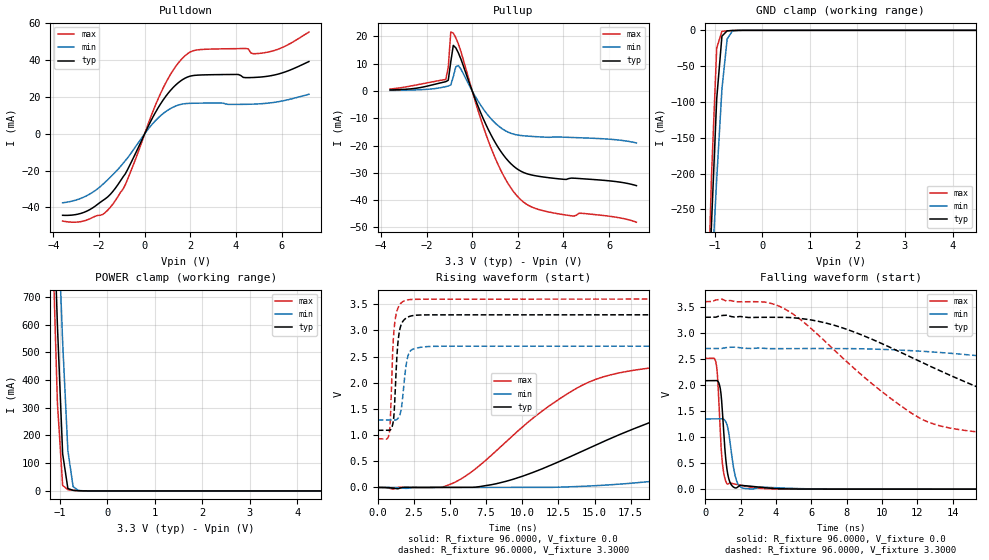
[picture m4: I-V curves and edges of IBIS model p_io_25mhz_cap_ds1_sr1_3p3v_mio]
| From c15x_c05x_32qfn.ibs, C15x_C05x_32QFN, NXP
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[Model] p_io_25mhz_cap_ds1_sr1_3p3v_mio
|   Model p_io_25mhz_cap_ds1_sr1_3p3v_mio
| This model was characterised for following simulation conditions:
| External (pad) voltage:
|   - Typ: 3.3V,   - Min: 2.7V,   - Max: 3.6V
| Library cells for typ/min/max conditions are connected as defined below:
|  pad - External Pad
|  ipp_do_lv - Core Input
|  ipp_obe_lv - Output Buffer Enable
|  IOGC - NC
|  REFH3V3 - REFH3V3
|  REFL3V3 - REFL3V3
|  ZI - NC
|  abut_ncal_vddio[1] - vddio
|  abut_ncal_vddio[2] - vddio
|  abut_ncal_vddio[3] - vssio
|  abut_ncal_vddio[4] - vddio
|  abut_ncal_vddio[5] - vddio
|  abut_ncal_vddio[6] - vssio
|  abut_pcal_vddio[1] - vssio
|  abut_pcal_vddio[2] - vssio
|  abut_pcal_vddio[3] - vddio
|  abut_pcal_vddio[4] - vssio
|  abut_pcal_vddio[5] - vssio
|  abut_pcal_vddio[6] - vddio
|  ipp_do_1p8v - ipp_do_1p8v
|  ipp_dse_lv - vdd_lv
|  ipp_eftd_lv - NC
|  ipp_ina_mux_vddio - NC
|  ipp_ina_mux_vddio[0] - NC
|  ipp_ina_mux_vddio[1] - NC
|  ipp_ina_r0_vddio - NC
|  ipp_ina_r0a_vddio - NC
|  ipp_ina_r0b_vddio - NC
|  ipp_ina_r0c_vddio - NC
|  ipp_ina_r0d_vddio - NC
|  ipp_ina_r0e_vddio - NC
|  ipp_ina_r0f_vddio - NC
|  ipp_ina_r300_vddio - NC
|  ipp_ina_r300a_vddio - NC
|  ipp_ina_r300b_vddio - NC
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Model_type I/O
Polarity   Non-Inverting
Enable   Active-High
Vinl =   0.9900V
Vinh =   2.3100V
Vmeas =  1.6500V
Cref =   30.0000pF
Rref =   1.0000M
Vref =   3.3000V
C_comp   1.2811pF   1.2304pF   1.3502pF
|C_comp_pullup   0.5378pF   0.5690pF   0.5165pF
|C_comp_pulldown   0.6572pF   0.6938pF   0.6280pF
[Model Spec]
| variable   typ   min   max
Vinh   2.3100V   1.8900V   2.5200V
Vinl   0.9900V   0.8100V   1.0800V
[Temperature Range]   25.0000   0.1250k   -40.0000
[Voltage Range]   3.3000V   2.7000V   3.6000V
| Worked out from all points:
|   slope of the pulldown table from 0 to 0.495 V, typ, clamps not added: 40.8 ohm
|   slope of the pullup table from 0 to 0.495 V, typ, clamps not added: 47.8 ohm
|   GND clamp passes 1 mA (typ) near -0.74 V on its own axis
|   POWER clamp passes 1 mA (typ) near -0.62 V on its own axis
|   rising waveform, R_fixture 96.0000, V_fixture 0.0: 20-80 % time 12ns typ, 25.5ns min, 7.17ns max; typ from 0 V to 2.08 V
|   rising waveform, R_fixture 96.0000, V_fixture 3.3000: 20-80 % time 277ps typ, 348ps min, 248ps max; typ from 1.09 V to 3.3 V
|   falling waveform, R_fixture 96.0000, V_fixture 0.0: 20-80 % time 280ps typ, 355ps min, 248ps max; typ from 2.08 V to 0 V
|   falling waveform, R_fixture 96.0000, V_fixture 3.3000: 20-80 % time 9.25ns typ, 20.1ns min, 5.6ns max; typ from 3.3 V to 1.09 V
[Pulldown]
|Voltage   I(typ)   I(min)   I(max)
-3.6V     -44.37mA   -37.58mA   -47.51mA
-2.5V     -41.88mA   -33.45mA   -46.76mA
-1.84V    -36.35mA   -27.58mA   -43.93mA
-1.4V     -31.44mA   -22.29mA   -38.35mA
-850mV    -21.79mA   -14.63mA   -27.74mA
800mV     18.21mA    10.89mA    24.66mA
1.35V     26.41mA    15.03mA    36.45mA
1.9V      30.96mA    16.49mA    43.73mA
4.43V     30.52mA    16mA       46.39mA
4.76V     30.6mA     16.11mA    43.53mA
5.31V     31.15mA    16.53mA    44.19mA
7.2V      39.28mA    21.46mA    55.3mA
[Pullup]
|Voltage   I(typ)   I(min)   I(max)
-3.6V     375uA      207.1uA    721uA
-1.16V    3.419mA    1.608mA    4.218mA
-1.05V    3.929mA    1.825mA    8.684mA
-940mV    10.66mA    2.209mA    21.58mA
-830mV    16.7mA     5.227mA    21.23mA
-720mV    15.82mA    8.86mA     19.48mA
-610mV    14mA       9.299mA    17.3mA
820mV     -16.02mA   -10.13mA   -20.76mA
1.48V     -24.66mA   -14.68mA   -32.62mA
2.03V     -28.88mA   -16.19mA   -39.03mA
3.35V     -31.76mA   -16.97mA   -44.31mA
7.2V      -34.67mA   -19.04mA   -48.06mA
[GND_clamp]
|Voltage   I(typ)   I(min)   I(max)
-3.6V     -5.309A    -4.128A    -6.876A
-1.18V    -466mA     -495.4mA   -458.9mA
-1.07V    -271.1mA   -348.5mA   -204.6mA
-960mV    -95.65mA   -207.9mA   -24.72mA
-850mV    -8.088mA   -81.85mA   -1.461mA
-740mV    -716.3uA   -12.13mA   -715.9uA
-630mV    -272.3uA   -921.7uA   -303uA
-300mV    -444.9nA   -2.656uA   -94.82nA
7.2V      0A         0A         0A
[POWER_clamp]
|Voltage   I(typ)   I(min)   I(max)
-3.6V     14.48A     12.95A     16.35A
-1.16V    1.177A     1.535A     951.2mA
-1.05V    598.4mA    1.032A     318mA
-940mV    134.2mA    537.3mA    20.05mA
-830mV    8.719mA    145.4mA    4.267mA
-720mV    2.135mA    15.38mA    2.236mA
-610mV    852.8uA    1.854mA    844.7uA
7.2V      0A         0A         0A
[Ramp]
| variable   typ   min   max
dV/dt_r  1.2491/12.0202n   0.8026/25.5328n   1.5061/7.1681n
dV/dt_f  1.3249/9.2464n   0.8437/20.0812n   1.6024/5.6024n
R_load = 96.0000
[Rising Waveform]
R_fixture= 96.0000
V_fixture= 0.0
V_fixture_min= 0.0
V_fixture_max= 0.0
|time   V(typ)   V(min)   V(max)
0s        3.103nV    104.7nV    10.53nV
4.6ns     -77.76uV   -441.7uV   17.67mV
8.624ns   98.53mV    14.04uV    808.3mV
11.42ns   360.6mV    557.1uV    1.468V
14.6ns    749.1mV    26.49mV    2.012V
21.81ns   1.523V     200.5mV    2.358V
31.45ns   1.89V      551.3mV    2.458V
42.94ns   2.004V     940.6mV    2.493V
53.91ns   2.045V     1.131V     2.504V
127.4ns   2.082V     1.338V     2.51V
[Rising Waveform]
R_fixture= 96.0000
V_fixture= 3.3000
V_fixture_min= 2.7000
V_fixture_max= 3.6000
|time   V(typ)   V(min)   V(max)
0s        1.092V     1.289V     929.3mV
800.7ps   1.091V     1.289V     1.05V
873ps     1.1V       1.289V     1.317V
1.02ns    1.189V     1.289V     2.533V
1.097ns   1.319V     1.289V     2.921V
1.293ns   2.363V     1.295V     3.34V
1.57ns    3.071V     1.429V     3.511V
1.974ns   3.239V     2.359V     3.58V
2.283ns   3.276V     2.616V     3.592V
127.4ns   3.3V       2.7V       3.6V
[Falling Waveform]
R_fixture= 96.0000
V_fixture= 0.0
V_fixture_min= 0.0
V_fixture_max= 0.0
|time   V(typ)   V(min)   V(max)
0s        2.082V     1.348V     2.51V
620.5ps   2.085V     1.348V     2.399V
703.3ps   2.075V     1.348V     2.108V
935.1ps   1.653V     1.351V     619.5mV
1.182ns   500.1mV    1.277V     131.2mV
1.426ns   110.4mV    836.6mV    119.3mV
1.649ns   29.61mV    322.9mV    99.39mV
1.858ns   46.57mV    95.2mV     85.86mV
3.317ns   27.55mV    37.09mV    11.46mV
127.4ns   207.7nV    4.321uV    21.7nV
[Falling Waveform]
R_fixture= 96.0000
V_fixture= 3.3000
V_fixture_min= 2.7000
V_fixture_max= 3.6000
|time   V(typ)   V(min)   V(max)
0s        3.3V       2.7V       3.6V
4.24ns    3.299V     2.698V     3.503V
7.731ns   3.101V     2.699V     2.534V
12.02ns   2.473V     2.652V     1.386V
17.37ns   1.698V     2.491V     1.044V
20.25ns   1.425V     2.368V     999.4mV
25.2ns    1.262V     2.132V     962.9mV
35.45ns   1.154V     1.676V     938.8mV
45.6ns    1.119V     1.478V     932.6mV
127.4ns   1.092V     1.294V     929.3mV
